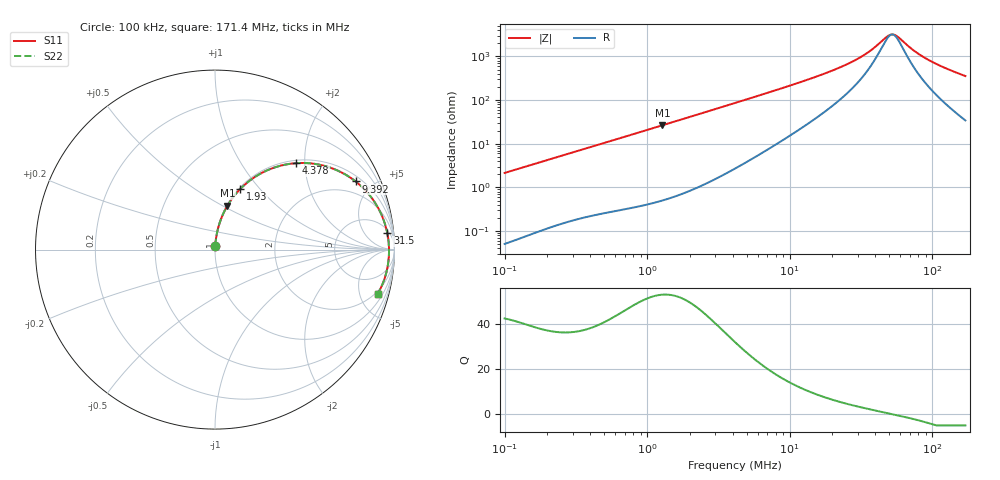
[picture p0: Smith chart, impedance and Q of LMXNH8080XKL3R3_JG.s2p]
! LMXNH8080XKL3R3_JG  S-PARAMETER MODEL  ( General Type )
! Model Generated by TAIYO YUDEN Corporation (http://www.ty-top.com)
! Version 1.0
! TAIYO YUDEN Control No. 191025NI43SB-FBB
! Copyright(c) 2019 TAIYO YUDEN CO.,LTD. All Rights Reserved.
! Product Description (link to TY-COMPAS)
! https://ds.yuden.co.jp/TYCOMPAS/or/detail?pn=LMXNH8080XKL3R3MJG&u=M
! Products Name : Inductors
! Characteristics :
!  Inductance : 3.3 uH , SRF(min) : 50 MHz , DC Resistance(max) : 0.0247 Ohm
!  Rated Current : Saturation :4200 mA , Temp Rise : 4300 mA
!  Case Size : 8.0 x 8.0 / 0.315 x 0.315 [mm/inch] , Thickness : 3 / 0.118 [mm/inch]
!  (Conditions: Temperature = 25 degC , DC Bias Current/Voltage = 0A / 0V)
! External Node Assignments :
!  1  o---GGG---o  2
! GND o---------o GND
! Frequency Range : 0.1MHz  -  171.398534MHz  [ 402 STEP ]
# MHz S RI R 50
! Freq[MHz].  S11 Real  S11 Imag  S21 Real  S21 Imag  S12 Real  S12 Imag  S22 Real  S22 Imag
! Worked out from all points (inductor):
!   401 points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, 100 kHz to 171.4 MHz, reference 50 ohm
!   read as one part in series: L = 3.4 uH near 103.8 kHz
!   highest Q = 52.8 at 1.281 MHz (marker M1), where L = 3.29 uH
!   self-resonance near 52.48 MHz
!   S11 on the Smith chart (normalised r, x): 100 kHz: 1.00, +0.04; 1.93 MHz: 1.02, +0.80; 4.378 MHz: 1.06, +1.81; 9.392 MHz: 1.27, +3.98; 31.5 MHz: 7, +18; 171.4 MHz: 1.68, -7.07
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0.1  0.000966 0.0214  0.999 -0.0214  0.999 -0.0214  0.000966 0.0214
0.348094  0.00724 0.0723  0.9928 -0.0723  0.9928 -0.0723  0.00724 0.0723
0.680388  0.0224 0.1375  0.9776 -0.1375  0.9776 -0.1375  0.0224 0.1375
1.211692  0.0629 0.2334  0.9371 -0.2334  0.9371 -0.2334  0.0629 0.2334
1.28129  0.0695 0.245  0.9305 -0.245  0.9305 -0.245  0.0695 0.245
1.929825  0.1419 0.3391  0.8581 -0.3391  0.8581 -0.3391  0.1419 0.3391
2.800388  0.2559 0.4246  0.7441 -0.4246  0.7441 -0.4246  0.2559 0.4246
4.140031  0.4263 0.4791  0.5737 -0.4791  0.5737 -0.4791  0.4263 0.4791
4.377827  0.4534 0.4817  0.5466 -0.4817  0.5466 -0.4817  0.4534 0.4817
6.235538  0.6235 0.4626  0.3765 -0.4626  0.3765 -0.4626  0.6235 0.4626
9.391703  0.7839 0.3795  0.2161 -0.3795  0.2161 -0.3795  0.7839 0.3795
14.41119  0.8874 0.2677  0.1126 -0.2677  0.1126 -0.2677  0.8874 0.2677
22.52891  0.9411 0.1604  0.0589 -0.1604  0.0589 -0.1604  0.9411 0.1604
31.49709  0.96 0.0919  0.04 -0.0919  0.04 -0.0919  0.96 0.0919
37.24223  0.9652 0.0607  0.0348 -0.0607  0.0348 -0.0607  0.9652 0.0607
50.16444  0.9694 0.00787  0.0306 -0.00787  0.0306 -0.00787  0.9694 0.00787
53.0458  0.9696 -0.00189  0.0304 0.00189  0.0304 0.00189  0.9696 -0.00189
56.09266  0.9696 -0.0117  0.0304 0.0117  0.0304 0.0117  0.9696 -0.0117
75.55554  0.9662 -0.0653  0.0338 0.0653  0.0338 0.0653  0.9662 -0.0653
98.05203  0.9574 -0.1163  0.0426 0.1163  0.0426 0.1163  0.9574 -0.1163
129.6379  0.939 -0.1777  0.061 0.1777  0.061 0.1777  0.939 -0.1777
171.3985  0.9062 -0.2472  0.0938 0.2472  0.0938 0.2472  0.9062 -0.2472
